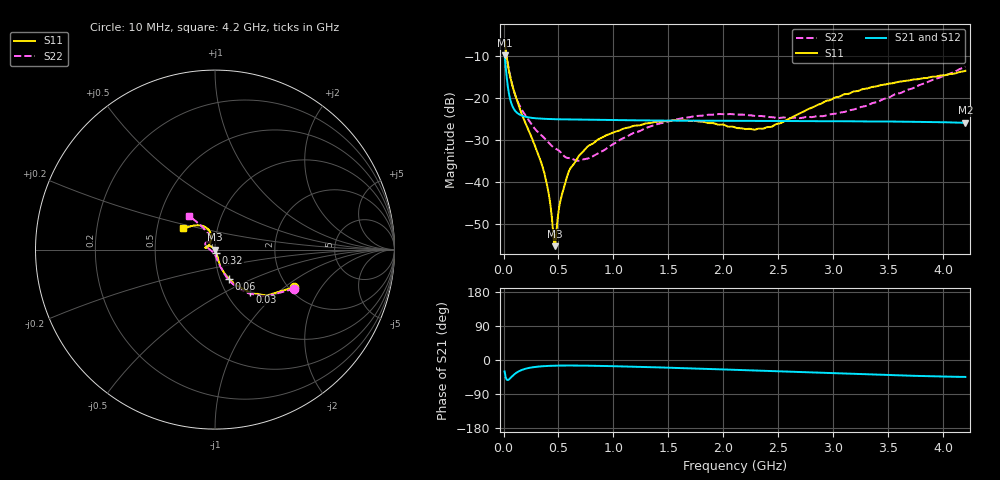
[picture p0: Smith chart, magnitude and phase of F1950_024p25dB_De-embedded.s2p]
! Integrated Device Technology
! Corporate Headquarters
! 6024 Silver Creek Valley Road
! San Jose, CA 95138  USA
! Phone:  1-408-284-8200
! Toll Free:  1-800-223-1366
! Webpage:  http://www.idt.com/
! Timing and RF Division
! 515 Groton Road, Suite 102
! Westford, MA 01886-6024
! Device:  F1950
! Description: 7-bit 0.25 dB Digital Step Attenuator
! Frequency:  150.0 -  4000.00 MHz
! Package:  4x4 mm Thin QFN Plastic Package: 24 pin
! Ports:  2 RF, 12 DC
!  Pin  1  = D0
!  Pin  2  = VDD
!  Pin  3  = Vmode
!  Pin  4  = GND
!  Pin  5  = RF1  =  Port 1
!  Pin  6  = GND
!  Pin  7  = GND
!  Pin  8  = GND
!  Pin  9  = GND
!  Pin 10  = GND
!  Pin 11  = GND
!  Pin 12  = GND
!  Pin 13  = GND
!  Pin 14  = RF2  =  Port 2
!  Pin 15  = GND
!  Pin 16  = LE
!  Pin 17  = CLK
!  Pin 18  = DATE
!  Pin 19  = D6
!  Pin 20  = D5
!  Pin 21  = D4
!  Pin 22  = D3
!  Pin 23  = D2
!  Pin 24  = D1
! State:  97
! Atten State:  24.25 dB
! Voltage:  +5.00 Volts
! Current:  Not Measured mA
! Data:  The device was measured on a the F195X evaluation board which has
!  individual transmission lines to the RF pins.  Data was collected
!  using a calibrated network analyzer.  The evaluation board was
!  de-embedded using a TRL calibration technique.
!  The reference plane is the edge of the package pin.
! Misc:  Board 2019
!  Action Tracker AT0250
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# GHz S dB R 50
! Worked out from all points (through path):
!   420 points, 10 MHz to 4.2 GHz, reference 50 ohm
!   highest |S21| = -9.69 dB at 10 MHz (marker M1); lowest = -25.9 dB at 4.2 GHz (marker M2)
!   group delay of S21, straight-line fit = 18.6 ps
!   lowest |S11| = -55.4 dB at 470 MHz (marker M3), VSWR 1.00, Z = 49.8 - j0.0374 ohm
!   |S11| at or under -10 dB: 28.62 MHz to end of sweep
!   |S22| runs from -34.9 to -6.2 dB; largest |S21 - S12| = 0.00012
!   S11 on the Smith chart (normalised r, x): 10 MHz: 2.14, -1.18; 30 MHz: 1.28, -0.67; 60 MHz: 1.11, -0.37; 320 MHz: 1.01, -0.04; 4.2 GHz: 0.68, +0.17
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0.01  -6.22 -25.3  -9.69 -30.3  -9.69 -30.3  -6.17 -26.3
0.03  -10.27 -51.0  -15.19 -52.2  -15.19 -52.2  -10.22 -52.4
0.06  -14.81 -64.0  -20.20 -48.6  -20.20 -48.6  -14.60 -65.5
0.1  -18.70 -70.6  -22.80 -37.4  -22.80 -37.4  -18.70 -70.9
0.15  -22.64 -72.4  -23.96 -28.3  -23.95 -28.3  -21.96 -75.0
0.32  -33.72 -71.4  -24.85 -17.3  -24.85 -17.3  -28.27 -83.6
0.39  -40.10 -71.6  -24.94 -15.8  -24.94 -15.9  -30.04 -86.6
0.42  -44.28 -79.1  -24.97 -15.4  -24.97 -15.5  -30.89 -88.7
0.45  -51.57 -101.5  -25.00 -15.1  -25.00 -15.1  -31.64 -93.1
0.47  -55.40 -167.2  -25.01 -15.0  -25.01 -15.0  -31.98 -96.4
0.48  -52.34 164.3  -25.02 -14.9  -25.02 -14.9  -32.14 -97.6
0.52  -44.22 143.3  -25.04 -14.7  -25.05 -14.7  -32.92 -100.9
0.58  -38.56 136.4  -25.07 -14.6  -25.07 -14.6  -34.27 -112.9
0.71  -33.10 138.8  -25.13 -14.8  -25.13 -14.8  -34.71 -137.8
1  -28.16 148.6  -25.23 -16.4  -25.23 -16.4  -30.94 -179.7
1.41  -25.62 163.8  -25.32 -19.5  -25.33 -19.5  -26.10 161.2
1.73  -25.38 169.3  -25.37 -22.2  -25.36 -22.2  -24.31 152.7
2.11  -27.03 159.3  -25.42 -26.1  -25.42 -26.1  -23.90 142.9
2.43  -26.86 127.7  -25.44 -28.9  -25.44 -29.0  -24.49 132.3
2.81  -22.19 106.1  -25.47 -33.0  -25.47 -33.0  -24.50 117.0
3.51  -16.47 118.0  -25.56 -39.9  -25.55 -39.9  -19.77 114.0
4.2  -13.44 146.1  -25.87 -44.7  -25.87 -44.7  -12.45 127.5
